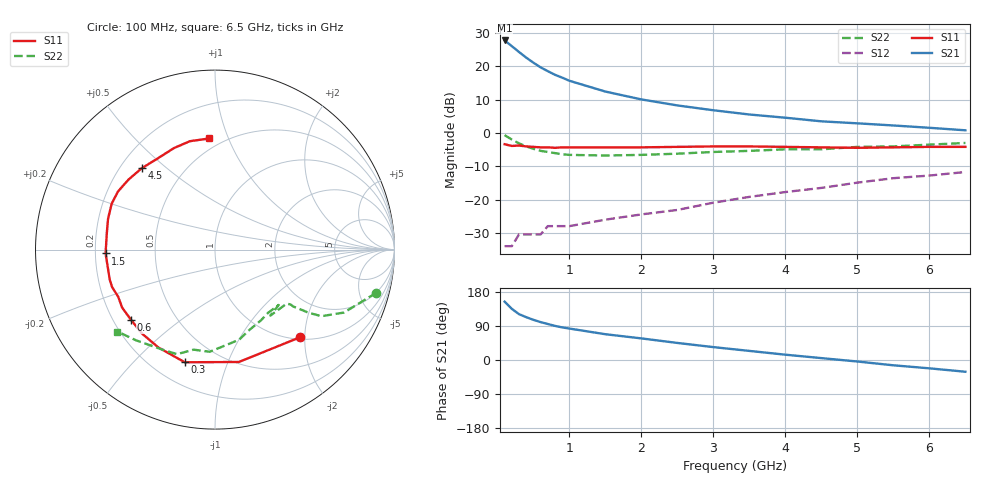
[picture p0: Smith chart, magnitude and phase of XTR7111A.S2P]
! HXTR-7111 Common Emitter
! Vce=10V  Ic=10mA
# ghz s ma r 50
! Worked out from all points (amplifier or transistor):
!   21 points, 100 MHz to 6.5 GHz, reference 50 ohm
!   highest |S21| = 27.8 dB at 100 MHz (marker M1)
!   |S21| within 3 dB of that: start of sweep to 273.3 MHz
!   unconditionally stable (mu >= 1): 1.458 GHz to 2.706 GHz
!   at 400 MHz: K = 0.39, MSG = 26.6 dB, |S12| = -30.5 dB
!   at 1.5 GHz: K = 1.01, MAG = 18.6 dB, |S12| = -26.0 dB
!   at 6.5 GHz: K = 0.41, MSG = 6.3 dB, |S12| = -11.7 dB
!   S11 on the Smith chart (normalised r, x): 100 MHz: 1.04, -1.89; 300 MHz: 0.33, -0.71; 600 MHz: 0.27, -0.34; 1.5 GHz: 0.24, -0.02; 4.5 GHz: 0.29, +0.41; 6.5 GHz: 0.42, +0.85
0.1  0.68 -46.0  24.6 154.0  0.02 63.0  0.93 -15.0
0.2  0.64 -78.0  20.2 135.0  0.02 56.0  0.8 -26.0
0.3  0.65 -105.0  16.5 121.0  0.03 47.0  0.7 -32.0
0.4  0.63 -120.0  13.6 113.0  0.03 43.0  0.63 -34.0
0.5  0.62 -131.0  11.4 106.0  0.03 39.0  0.58 -35.0
0.6  0.61 -140.0  9.7 100.0  0.03 43.0  0.54 -36.0
0.7  0.61 -148.0  8.5 95.0  0.04 43.0  0.52 -36.0
0.8  0.6 -154.0  7.5 90.0  0.04 43.0  0.5 -37.0
0.9  0.61 -160.0  6.8 86.0  0.04 43.0  0.48 -50.0
1  0.61 -164.0  6.1 83.0  0.04 43.0  0.47 -41.0
1.5  0.61 -178.0  4.2 68.0  0.05 49.0  0.46 -50.0
2  0.61 171.0  3.2 57.0  0.06 56.0  0.47 -57.0
2.5  0.62 164.0  2.6 45.0  0.07 60.0  0.49 -68.0
3  0.63 156.0  2.2 34.0  0.09 61.0  0.52 -75.0
3.5  0.63 149.0  1.9 24.0  0.11 61.0  0.54 -85.0
4  0.62 141.0  1.7 14.0  0.13 59.0  0.57 -93.0
4.5  0.61 132.0  1.5 5.0  0.15 57.0  0.57 -102.0
5  0.6 123.0  1.4 -4.0  0.18 53.0  0.62 -110.0
5.5  0.61 112.0  1.3 -14.0  0.21 48.0  0.63 -118.0
6  0.62 103.0  1.2 -22.0  0.23 43.0  0.67 -131.0
6.5  0.62 93.0  1.1 -31.0  0.26 36.0  0.71 -140.0
